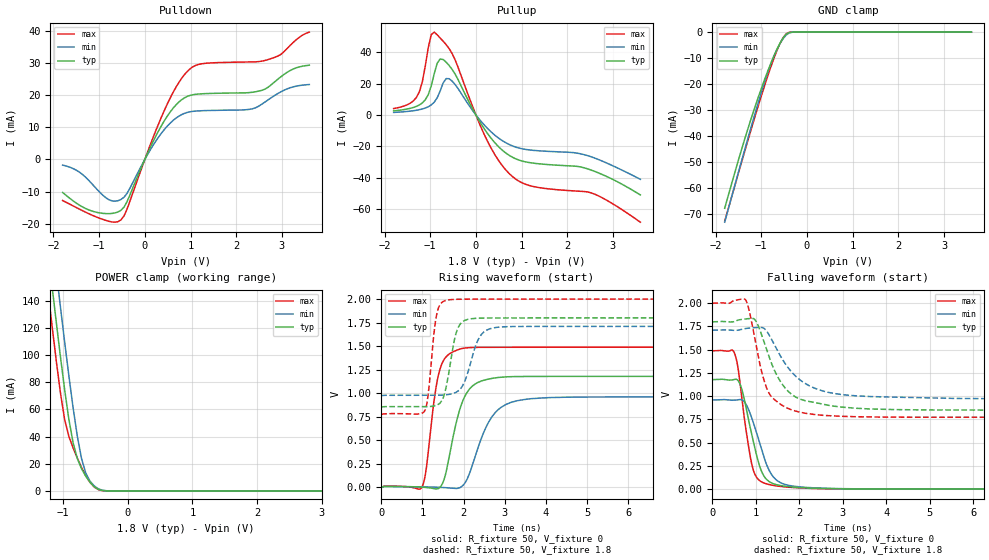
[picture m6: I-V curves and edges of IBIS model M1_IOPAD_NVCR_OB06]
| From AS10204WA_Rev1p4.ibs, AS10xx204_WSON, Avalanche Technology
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[Model] M1_IOPAD_NVCR_OB06
Model_type I/O
Enable   Active-High
Vinl  =  0.54
Vinh  =  1.26
Vmeas =  0.9
Cref  =  30e-12
| Capacitance  typ   min   max
C_comp   3.869840e-12   3.575244e-12   4.208825e-12
| Variables   typ   min   max
[GND Clamp Reference]   0   0   0
[POWER Clamp Reference]   1.8   1.71   2
[Pulldown Reference]   0   0   0
[Pullup Reference]   1.8   1.71   2
[Temperature Range]   25   105   -40
[Voltage Range]   1.8   1.71   2
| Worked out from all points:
|   slope of the pulldown table from 0 to 0.27 V, typ, clamps not added: 33.5 ohm
|   slope of the pullup table from 0 to 0.27 V, typ, clamps not added: 21.7 ohm
|   GND clamp passes 1 mA (typ) near -0.46 V on its own axis
|   POWER clamp passes 1 mA (typ) near -0.44 V on its own axis
|   falling waveform, R_fixture 50, V_fixture 0: 20-80 % time 349ps typ, 413ps min, 269ps max; typ from 1.18 V to 0 V
|   falling waveform, R_fixture 50, V_fixture 1.8: 20-80 % time 603ps typ, 781ps min, 399ps max; typ from 1.8 V to 0.85 V
|   rising waveform, R_fixture 50, V_fixture 0: 20-80 % time 395ps typ, 541ps min, 266ps max; typ from 0 V to 1.18 V
|   rising waveform, R_fixture 50, V_fixture 1.8: 20-80 % time 237ps typ, 326ps min, 166ps max; typ from 0.85 V to 1.8 V
[GND Clamp]
| Voltage   I(typ)   I(min)   I(max)
-1.8V     -67.84mA   -73.19mA   -72.81mA
-1.499V   -49.26mA   -53.93mA   -54.28mA
-1.303V   -37.87mA   -41.64mA   -42.4mA
-1.108V   -27.29mA   -29.68mA   -30.84mA
-912.4mV  -17.6mA    -18.46mA   -19.84mA
-782.1mV  -11.7mA    -11.87mA   -13.01mA
-651.7mV  -6.447mA   -6.494mA   -6.896mA
-521.4mV  -2.255mA   -2.526mA   -2.141mA
-456.2mV  -849.3uA   -1.156mA   -679.4uA
-391mV    -172uA     -356.5uA   -88.88uA
-260.7mV  -2.088uA   -12.98uA   -254.3nA
3.6V      0A         0A         0A
[POWER Clamp]
| Voltage   I(typ)   I(min)   I(max)
-1.8V     419.8mA    456.6mA    390.9mA
-1.238V   178mA      215.7mA    148.4mA
-1.173V   151mA      188.6mA    121.7mA
-1.108V   124.5mA    161.8mA    96mA
-1.043V   98.85mA    135.4mA    72.14mA
-977.6mV  74.56mA    109.6mA    52.56mA
-912.4mV  52.76mA    84.78mA    40.16mA
-847.2mV  35.48mA    61.36mA    31.71mA
-716.9mV  16.42mA    23.91mA    17.31mA
-651.7mV  10.9mA     13.27mA    11.28mA
-456.2mV  1.168mA    1.554mA    921.1uA
3.6V      0A         0A         0A
[Pulldown]
| Voltage   I(typ)   I(min)   I(max)
-1.8V     -10.27mA   -1.775mA   -12.78mA
-1.108V   -16.27mA   -8.366mA   -17.63mA
-782.1mV  -16.86mA   -12.57mA   -19.26mA
-521.4mV  -15.81mA   -12.45mA   -18.8mA
-391mV    -13.18mA   -10.58mA   -15.51mA
372.4mV   10.72mA    8.327mA    13.47mA
931mV     19.6mA     14.61mA    27.38mA
1.241V    20.39mA    15.13mA    29.72mA
2.283V    20.76mA    15.55mA    30.29mA
2.697V    22.43mA    18.5mA     31.03mA
3.179V    27.62mA    22.27mA    35.42mA
3.6V      29.28mA    23.28mA    39.58mA
[Pullup]
| Voltage   I(typ)   I(min)   I(max)
-1.8V     2.579mA    1.61mA     4.066mA
-1.434V   4.243mA    2.446mA    7.556mA
-1.238V   6.367mA    3.341mA    14.71mA
-977.6mV  18.53mA    6.386mA    51.24mA
-912.4mV  26.3mA     8.148mA    52.93mA
-782.1mV  35.76mA    15.3mA     49.13mA
-586.6mV  31.61mA    23.14mA    42.42mA
248.3mV   -11.6mA    -8.437mA   -16.46mA
744.8mV   -26.1mA    -19.1mA    -37.9mA
1.241V    -30.74mA   -22.58mA   -45.62mA
2.559V    -35.62mA   -27.1mA    -50.14mA
3.6V      -51.1mA    -41.13mA   -68.52mA
[Ramp]
dV/dt_r   0.70702/0.39465n  0.575676/0.54071n  0.892904/0.26596n
dV/dt_f   0.569737/0.602924n  0.44258/0.781144n  0.736237/0.398943n
R_load = 50
[Falling Waveform]
R_fixture = 50
V_fixture = 0
V_fixture_min = 0
V_fixture_max = 0
| Time   V(typ)   V(min)   V(max)
0s        1.178V     959.5mV    1.488V
505.1ps   1.181V     956.9mV    1.468V
580.5ps   1.173V     961.7mV    1.331V
666.6ps   1.092V     962.8mV    1.026V
802.5ps   815.2mV    888.9mV    548.2mV
942.9ps   513.8mV    715.5mV    204.1mV
1.169ns   155.3mV    370.1mV    69.9mV
1.455ns   50.58mV    105.8mV    36.41mV
3.196ns   2.704mV    4.128mV    1.706mV
21.88ns   366.3nV    781.9nV    391.8nV
[Falling Waveform]
R_fixture = 50
V_fixture = 1.8
V_fixture_min = 1.71
V_fixture_max = 2
| Time   V(typ)   V(min)   V(max)
0s        1.8V       1.71V      2V
755.5ps   1.831V     1.727V     2.041V
844.1ps   1.835V     1.732V     1.927V
996.5ps   1.813V     1.738V     1.569V
1.16ns    1.624V     1.737V     1.217V
1.324ns   1.398V     1.644V     1.016V
1.745ns   1.052V     1.305V     867.5mV
2.335ns   934mV      1.089V     803.4mV
5.619ns   851.2mV    975.9mV    773.6mV
21.88ns   850.4mV    972.4mV    772.9mV
[Rising Waveform]
R_fixture = 50
V_fixture = 0
V_fixture_min = 0
V_fixture_max = 0
| Time   V(typ)   V(min)   V(max)
0s        82.33nV    382.9nV    142.2nV
973ps     173.1uV    2.959mV    -10.32mV
1.088ns   -3.879mV   2.206mV    184mV
1.28ns    -16.31mV   -58.62uV   915.4mV
1.431ns   279.3uV    -2.673mV   1.264V
1.556ns   128.3mV    -5.773mV   1.377V
1.99ns    928.5mV    21.95mV    1.477V
2.703ns   1.157V     758.1mV    1.487V
3.631ns   1.177V     940.1mV    1.488V
21.88ns   1.178V     959.5mV    1.488V
[Rising Waveform]
R_fixture = 50
V_fixture = 1.8
V_fixture_min = 1.71
V_fixture_max = 2
| Time   V(typ)   V(min)   V(max)
0s        850.4mV    972.4mV    772.9mV
1.064ns   854.1mV    975.9mV    819mV
1.134ns   855.2mV    975.5mV    971.4mV
1.336ns   869.6mV    975.3mV    1.817V
1.512ns   961.3mV    978.7mV    1.976V
1.639ns   1.214V     985.7mV    1.992V
1.926ns   1.739V     1.048V     1.998V
2.389ns   1.797V     1.597V     1.999V
2.88ns    1.799V     1.702V     1.999V
21.88ns   1.8V       1.71V      2V
